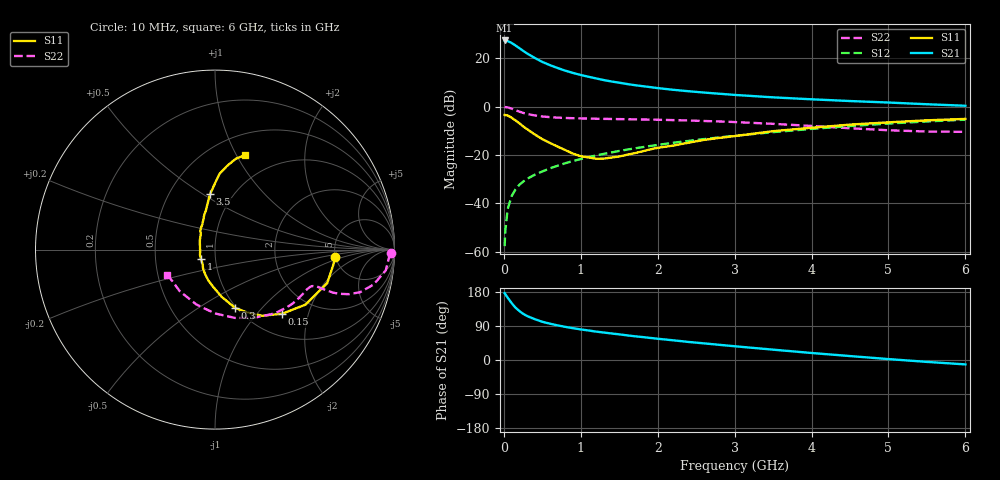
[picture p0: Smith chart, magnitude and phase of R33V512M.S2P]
! SIEMENS Small Signal Semiconductors
! BFR181
! Si NPN RF Bipolar Junction Transistor in SOT23
! VCE = 3.5 V  IC = 12 mA
! Common Emitter S-Parameters:  May  1996
# GHz  S  MA  R  50
!  f  S11  S21  S12  S22
! GHz  MAG  ANG  MAG  ANG  MAG  ANG  MAG  ANG
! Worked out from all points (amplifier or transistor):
!   36 points, 10 MHz to 6 GHz, reference 50 ohm
!   highest |S21| = 27.3 dB at 10 MHz (marker M1)
!   |S21| within 3 dB of that: start of sweep to 193.5 MHz
!   unconditionally stable (mu >= 1): 684.4 MHz to 2.583 GHz
!   at 250 MHz: K = 0.66, MSG = 27.1 dB, |S12| = -31.1 dB
!   at 1.4 GHz: K = 1.07, MAG = 13.1 dB, |S12| = -19.0 dB
!   at 6 GHz: K = 0.85, MSG = 2.9 dB, |S12| = -5.4 dB
!   S11 on the Smith chart (normalised r, x): 10 MHz: 4.92, -0.77; 150 MHz: 1.41, -1.38; 300 MHz: 0.99, -0.72; 1 GHz: 0.85, -0.09; 3.5 GHz: 0.79, +0.54; 6 GHz: 0.71, +1.09
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0.01  0.6689 -3.7  23.18 176.4  0.0013 84.4  0.9785 -1.2
0.02  0.666 -6.8  22.86 173.3  0.0028 79.0  0.9699 -2.8
0.05  0.6524 -16.7  22.46 164.4  0.0076 82.2  0.9586 -6.9
0.1  0.5895 -31.4  20.66 150.6  0.0139 78.1  0.9052 -12.4
0.15  0.5172 -43.7  18.32 138.4  0.0192 72.1  0.8421 -16.4
0.2  0.4529 -54.5  16.15 129.5  0.024 70.6  0.7865 -18.4
0.25  0.3906 -63.3  14.19 122.0  0.0279 69.3  0.7387 -19.5
0.3  0.3422 -71.1  12.55 116.2  0.0319 68.9  0.7031 -20.0
0.4  0.266 -81.9  10.12 108.0  0.0388 69.2  0.6547 -20.1
0.5  0.2116 -91.9  8.356 100.8  0.0455 69.9  0.6226 -20.0
0.6  0.1766 -101.9  7.151 95.8  0.0529 70.6  0.6028 -19.9
0.7  0.1482 -111.6  6.235 91.3  0.0599 71.4  0.5892 -20.2
0.8  0.1257 -121.9  5.497 87.4  0.0674 71.1  0.58 -20.5
1  0.0937 -147.8  4.487 80.7  0.0821 71.5  0.5678 -21.6
1.1  0.089 -160.7  4.122 77.9  0.0898 71.4  0.5629 -22.5
1.3  0.0839 174.2  3.519 72.5  0.1052 70.9  0.5551 -24.2
1.6  0.1009 146.3  2.92 65.0  0.1287 69.8  0.5466 -27.4
2.2  0.1556 117.2  2.218 52.0  0.178 66.4  0.5242 -35.5
3.5  0.3092 95.1  1.547 27.3  0.2953 55.6  0.4387 -59.9
4.5  0.4227 86.6  1.298 10.4  0.3951 44.5  0.3555 -90.1
5.5  0.5181 77.2  1.114 -5.0  0.4913 31.3  0.3038 -130.2
6  0.5546 72.3  1.037 -11.6  0.5347 24.1  0.2996 -152.3
